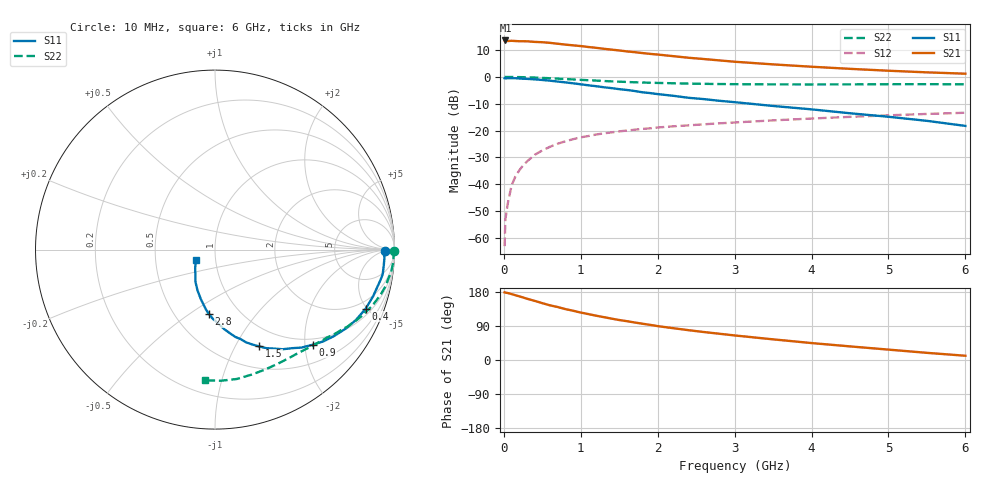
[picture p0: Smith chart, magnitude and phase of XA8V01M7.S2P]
! SIEMENS Discrete & RF Semiconductors
! BFY180
! Si NPN RF Bipolar Junction Transistor in MICRO-X
! VCE = 8 V  IC = 1.7 mA
! Common Emitter S-Parameters:  May  1997
# GHz  S  MA  R  50
!  f  S11  S21  S12  S22
! GHz  MAG  ANG  MAG  ANG  MAG  ANG  MAG  ANG
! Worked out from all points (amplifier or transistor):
!   36 points, 10 MHz to 6 GHz, reference 50 ohm
!   highest |S21| = 13.6 dB at 20 MHz (marker M1)
!   |S21| within 3 dB of that: start of sweep to 1.272 GHz
!   unconditionally stable (mu >= 1): 3.404 GHz to end of sweep
!   at 250 MHz: K = 0.09, MSG = 23.1 dB, |S12| = -33.0 dB
!   at 1.4 GHz: K = 0.59, MSG = 15.4 dB, |S12| = -20.7 dB
!   at 6 GHz: K = 1.05, MAG = 5.9 dB, |S12| = -13.4 dB
!   S11 on the Smith chart (normalised r, x): 10 MHz: 35, -4; 400 MHz: 1.40, -4.91; 900 MHz: 0.87, -2.17; 1.5 GHz: 0.75, -1.25; 2.8 GHz: 0.73, -0.60; 6 GHz: 0.80, -0.09
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0.01  0.9459 -0.4  4.757 178.5  0.0007 91.4  0.9975 -0.3
0.02  0.9402 -1.1  4.782 177.9  0.0022 96.7  0.9967 -0.6
0.05  0.9453 -2.7  4.666 176.8  0.0043 84.9  0.9957 -1.5
0.1  0.9444 -5.3  4.709 174.0  0.0094 86.1  0.9957 -3.0
0.15  0.9444 -8.4  4.667 171.0  0.0139 85.3  0.9943 -4.6
0.3  0.919 -16.3  4.613 161.8  0.0265 79.2  0.9808 -9.1
0.4  0.9017 -21.4  4.495 156.1  0.0352 76.2  0.9728 -11.9
0.5  0.8776 -26.6  4.434 150.0  0.0426 72.7  0.9589 -14.7
0.6  0.8505 -31.2  4.314 144.2  0.0499 69.6  0.9439 -17.3
0.9  0.7599 -44.2  3.879 130.0  0.0691 61.5  0.8976 -24.3
1  0.7288 -48.5  3.757 125.2  0.0748 59.1  0.8826 -26.3
1.1  0.697 -52.0  3.609 121.1  0.0791 57.1  0.8668 -28.2
1.2  0.6712 -55.8  3.485 116.9  0.0845 55.1  0.8536 -30.2
1.5  0.5918 -65.6  3.115 105.5  0.0966 50.2  0.8157 -35.2
1.8  0.5174 -74.2  2.786 95.8  0.1073 46.7  0.787 -39.5
2  0.4783 -79.3  2.612 89.4  0.1141 44.4  0.7725 -42.3
2.2  0.4453 -83.5  2.439 84.0  0.1199 42.2  0.7619 -45.1
2.8  0.3593 -95.5  2.033 69.3  0.1363 37.5  0.7366 -52.5
3.5  0.2874 -105.9  1.712 54.5  0.1549 32.1  0.7259 -61.0
4.5  0.2101 -121.2  1.414 35.9  0.1801 24.9  0.7258 -73.7
5.5  0.1518 -136.7  1.216 18.9  0.2041 17.3  0.7313 -87.3
6  0.1221 -151.9  1.148 11.2  0.2149 13.1  0.7303 -94.2
